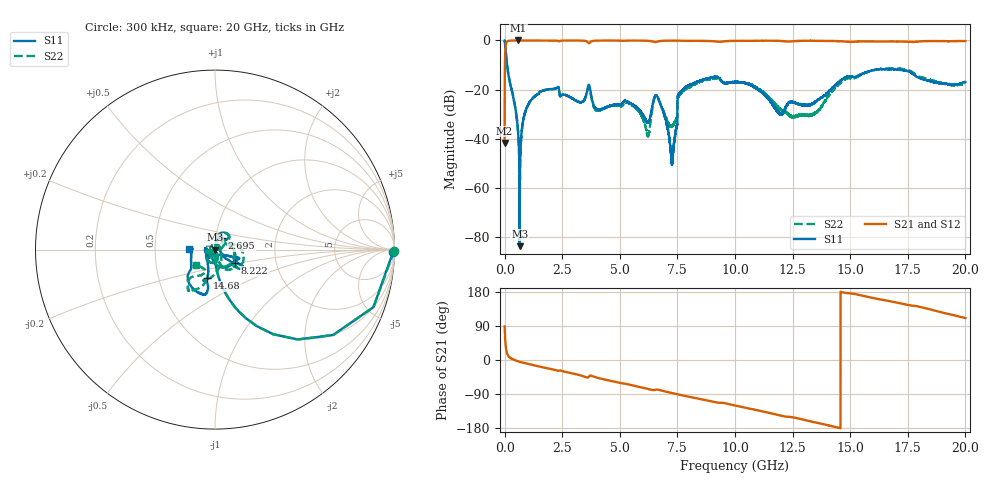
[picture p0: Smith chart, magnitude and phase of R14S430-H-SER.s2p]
!{R14S430}
!Johanson Technology Inc.
!www.johansontechnology.com
!Test Board Conditions:
!Substrate Type  RO4350B
!Substrate Thickness  20 mil
!Substrate Dk  3.66
!TL Type: GCPW
!TL Trace Width  36 mil
!TL Gap  12 mil
!Electrode orientation  Horizontal
!DUT TOPOLOGY	SERIES
!Mounting Pad LxW  26x36 mil
! Created Wed Nov 25 17:33:21 2020
! 2 Port Network Data from SP1.SP block
! freq  magS11  angS11  magS21  angS21  magS12  angS12  magS22  angS22
# khz S ma R 50
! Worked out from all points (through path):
!   20001 points, 300 kHz to 20 GHz, reference 50 ohm
!   highest |S21| = 0.00 dB at 594.3 MHz (marker M1); lowest = -41.7 dB at 300 kHz (marker M2)
!   group delay of S21, straight-line fit = 34.7 ps
!   lowest |S11| = -83.8 dB at 655.3 MHz (marker M3), VSWR 1.00, Z = 50 + j0.00368 ohm
!   |S11| at or under -10 dB: 107.2 MHz to end of sweep
!   |S22| runs from -68.6 to 0.0 dB; largest |S21 - S12| = 0.016
!   S11 on the Smith chart (normalised r, x): 300 kHz: open; 2.695 GHz: 1.07, +0.14; 8.222 GHz: 1.24, -0.19; 14.68 GHz: 0.87, -0.28; 20 GHz: 0.75, +0.00
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300  0.9927 -0.7  0.008187 88.5  0.008142 89.9  0.9967 -0.6
116300  0.2925 -73.7  0.9548 16.1  0.9551 16.1  0.2936 -73.7
594300  0.01179 -93.8  0.9999 -3.6  0.9991 -3.6  0.01209 -92.0
655300  6.452e-05 34.8  0.999 -4.7  0.9994 -4.7  0.0006272 -64.5
875300  0.03288 81.8  0.9992 -8.4  0.9984 -8.4  0.03235 80.3
1209300  0.06579 77.1  0.9964 -13.2  0.9966 -13.2  0.06533 75.7
2695300  0.07561 58.9  0.9937 -32.1  0.9936 -32.1  0.07545 55.0
3334300  0.05518 42.0  0.9913 -41.1  0.9918 -41.1  0.05467 44.6
3648300  0.1239 -29.2  0.8813 -45.0  0.8821 -45.0  0.1168 -28.3
4039300  0.03903 -116.4  0.9909 -47.2  0.9915 -47.2  0.03761 -142.9
5380300  0.05506 -135.1  0.9916 -64.6  0.9919 -64.6  0.05267 -166.1
6208300  0.02136 -105.7  0.9838 -76.1  0.985 -76.1  0.01177 -128.8
6667300  0.06611 -130.9  0.9562 -78.4  0.9561 -78.4  0.06527 -130.8
7270300  0.003357 101.2  0.9925 -87.3  0.9922 -87.3  0.01822 -87.0
7600300  0.084 -38.3  0.9881 -91.8  0.9879 -91.7  0.07789 27.0
8222300  0.1344 -33.9  0.9807 -99.5  0.9813 -99.4  0.1264 10.0
1.00003e7  0.1428 -19.8  0.9794 -120.1  0.9796 -120.1  0.1411 -45.9
1.19643e7  0.03208 -75.8  0.9787 -146.4  0.978 -146.3  0.04006 -81.7
1.33343e7  0.05064 -157.7  0.9833 -162.7  0.9837 -162.7  0.0301 9.6
1.46763e7  0.1636 -105.5  0.9567 178.6  0.9578 178.6  0.1502 -95.6
1.66673e7  0.2551 -108.1  0.9549 155.8  0.9473 155.6  0.2711 -122.3
2e7  0.1441 179.2  0.9722 110.6  0.971 110.7  0.1347 -142.2
